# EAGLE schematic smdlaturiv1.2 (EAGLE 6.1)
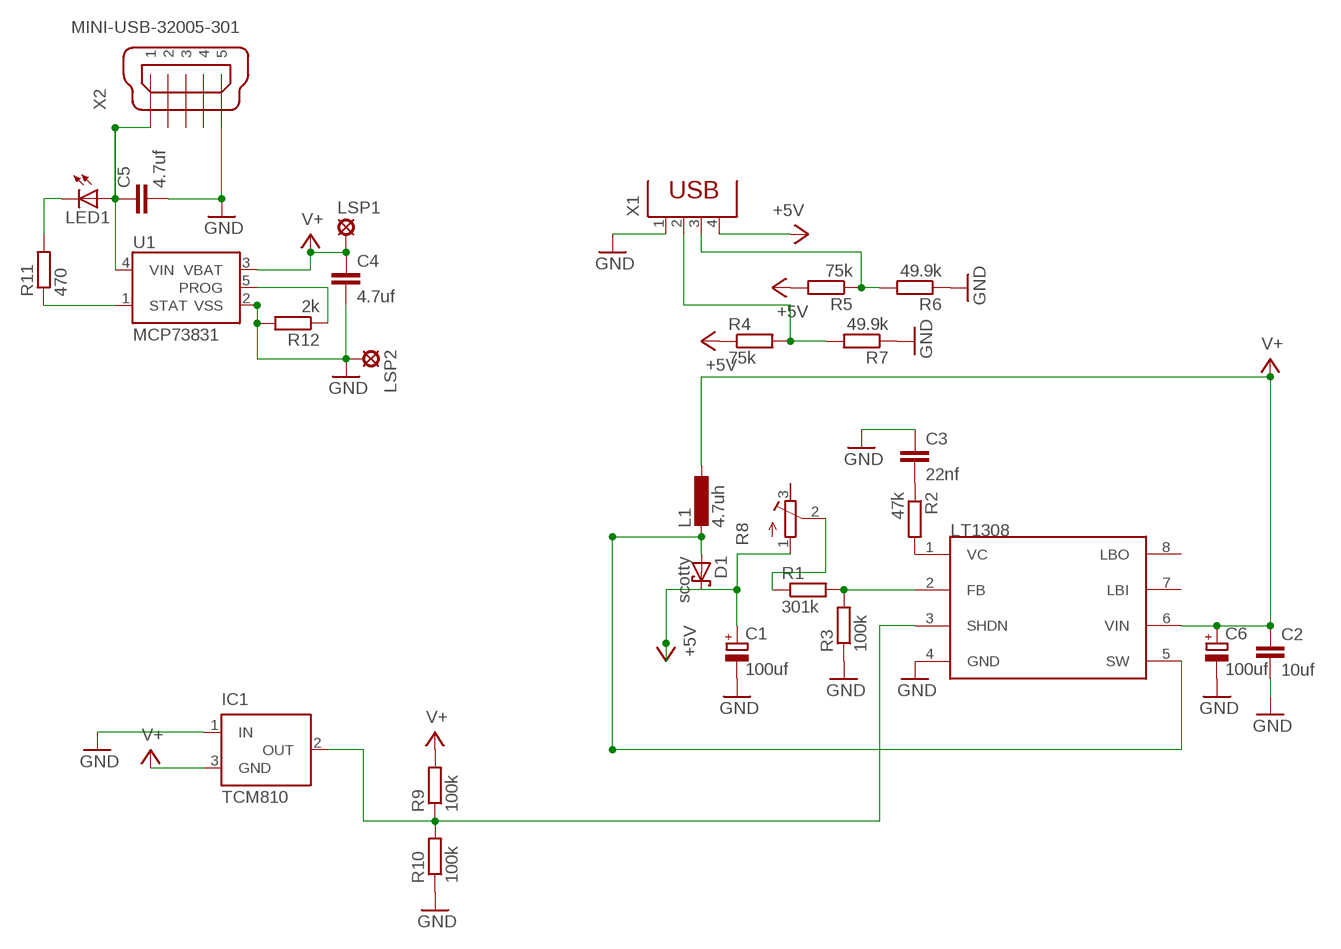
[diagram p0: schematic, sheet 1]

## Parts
C1  100uf  CPOL-EU153CLV-0605  [153CLV-0605]
C2  10uf  C-EUC1206  [C1206]
C3  22nf  C-EUC1206  [C1206]
C4  4.7uf  C-EUC1206  [C1206]
C5  4.7uf  C-EUC1206  [C1206]
C6  100uf  CPOL-EU153CLV-0605  [153CLV-0605]
D1  scotty  SCHOTTKY-DIODESMD  [SMB]
IC1  TCM810  MAX6520  [SOT23]
L1  4.7uh  L-EUL5038P  [L5038P]
LED1  LED3MM  [LED3MM]
LSP1  LSP10  [LSP10]
LSP2  LSP10  [LSP10]
R1  301k  R-EU_R1206  [R1206]
R2  47k  R-EU_R1206  [R1206]
R3  100k  R-EU_R1206  [R1206]
R4  75k  R-EU_R1206  [R1206]
R5  75k  R-EU_R1206  [R1206]
R6  49.9k  R-EU_R1206  [R1206]
R7  49.9k  R-EU_R1206  [R1206]
R8  R-TRIMM3103  [RTRIM3103]
R9  100k  R-EU_R1206  [R1206]
R10  100k  R-EU_R1206  [R1206]
R11  470  R-EU_R1206  [R1206]
R12  2k  R-EU_R1206  [R1206]
U1  MCP73831  [SOT23-5]
U$1  LT1308  [LT1308]
X1  PN87520  [PN87520]
X2  MINI-USB-32005-301  [32005-301]

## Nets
+5V: C1.+ D1.C R4.1 R5.2 R8.1(E) X1.4
GND: C1.- C2.2 C3.1 C4.2 C5.2 C6.- IC1.1(IN) LSP2.MP R3.1 R6.1 R7.1 R10.1 R12.2 U1.2(VSS) U$1.4(GND) X1.1 X2.5
N$1: R1.2 R3.2 U$1.2(FB)
N$2: R2.2 U$1.1(VC)
N$4: C3.2 R2.1
N$5: D1.A L1.2 U$1.5(SW)
N$6: R4.2 R7.2 X1.2
N$7: R5.1 R6.2 X1.3
N$11: IC1.2(OUT) R9.1 R10.2 U$1.3(SHDN)
N$13: R1.1 R8.2(S)
N$14: C5.1 LED1.A U1.4(VIN) X2.1
N$16: LED1.K(C) R11.2
N$17: R11.1 U1.1(STAT)
N$19: R12.1 U1.5(PROG)
V+: C2.1 C4.1 C6.+ IC1.3(GND) L1.1 LSP1.MP R9.2 U1.3(VBAT) U$1.6(VIN)
Unconnected: R8.3(A) U$1.7(LBI) U$1.8(LBO) X2.2 X2.3 X2.4

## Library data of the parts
C1 C6 = resistor:CPOL-EU: POLARIZED CAPACITOR, European symbol
C2-C5 = resistor:C-EU: CAPACITOR, European symbol
D1 = diode:SCHOTTKY-DIODE: Schottky Diode
IC1 = maxim:MAX6520: 1.2V Voltage Reference 50ppm/°C, SOT23, 3-Terminal Source: Data sheet; MF: MAXIM; MPN: MAX6520EUR-T; OC_FARNELL: unknown; OC_NEWARK: 02J4586
L1 = resistor:L-EU: INDUCTOR, European symbol
LED1 = led:LED: LED
LSP1 LSP2 = solpad:LSP10: SOLDER PAD
R1-R7 R9-R12 = resistor:R-EU_: RESISTOR, European symbol
R8 = resistor:R-TRIMM: Trimm resistor
U1 = SparkFun-PowerIC:MCP73831: Miniature single cell, fully integrated Li-Ion, Li-polymer charge management controller http://ww1.microchip.com/downloads/en/DeviceDoc/21984a.pdf
U$1 = lt1308:LT1308
X1 = con-berg:PN87520: BERG USB connector; OC_FARNELL: unknown; OC_NEWARK: unknown
X2 = con-cypressindustries:MINI-USB-: MINI USB-B Conector Source: www.cypressindustries.com; OC_FARNELL: unknown; OC_NEWARK: unknown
